PROGRAM AMCI_Assembled_Move_Sample
VAR
FB_Program_Assembled_Move: program_assembled_move_dut;
b_program_assembled_en: BOOL;
b_program_assembled_er: BOOL;
b_program_assembled_dn: BOOL;

FB_run_blend: run_blend_dut;
b_run_blend_en: BOOL;
b_run_blend_er: BOOL;

END_VAR
VAR // added by the converter: edge detectors and wires of the graphical bodies
    _w1, _w2 : BOOL;
END_VAR

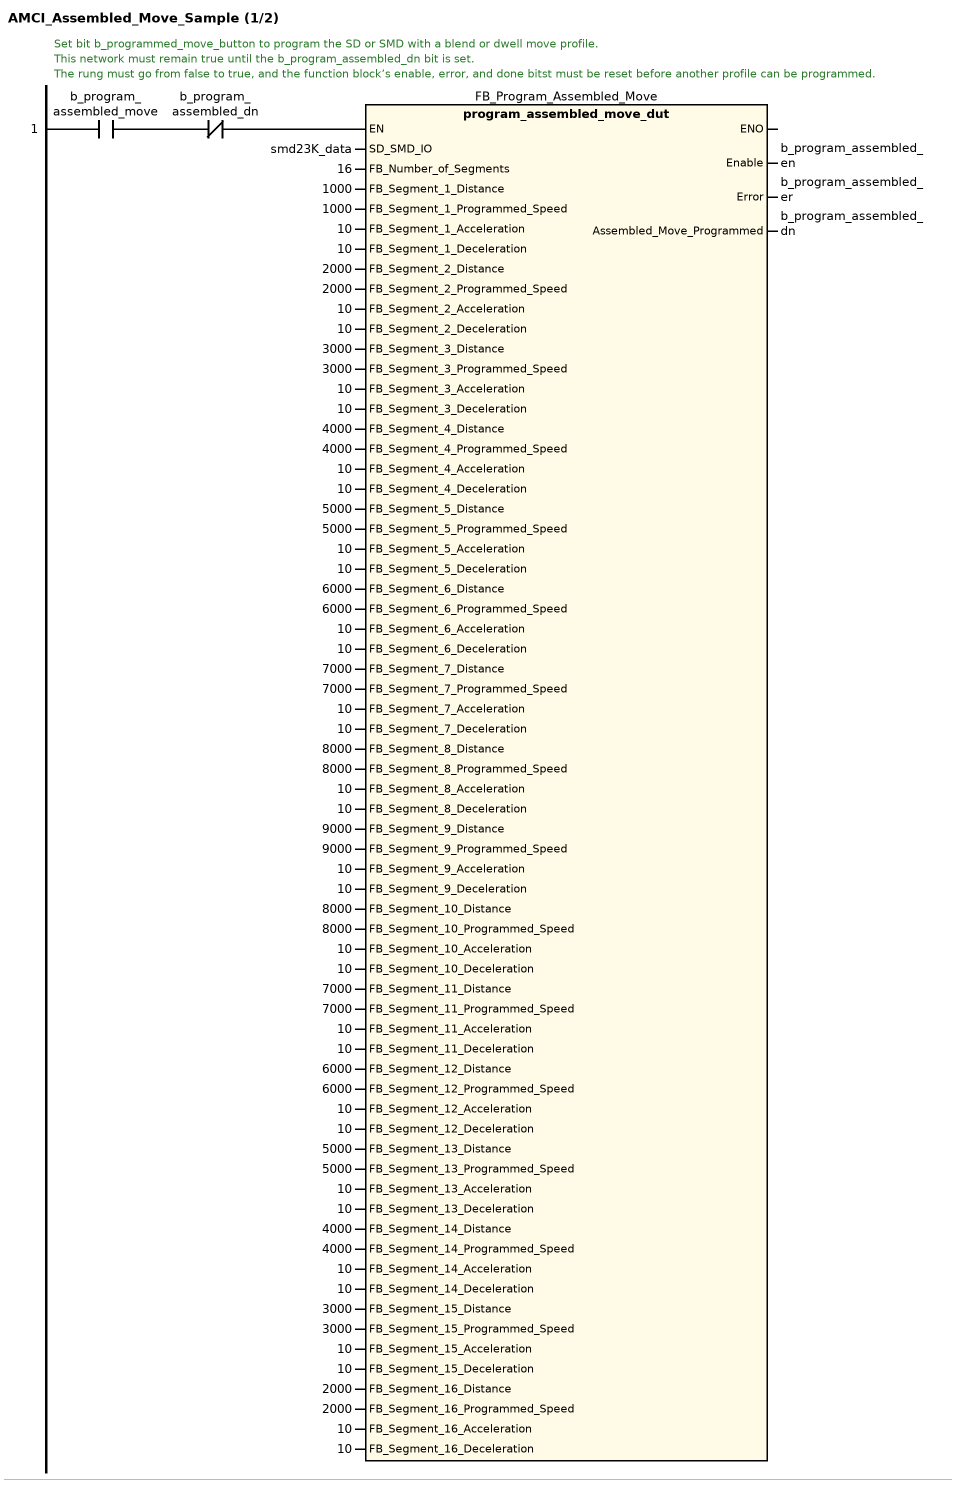
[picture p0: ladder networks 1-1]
// NETWORK 1
// Set bit b_programmed_move_button to program the SD or SMD with a blend or dwell move profile.
//
// This network must remain true until the b_program_assembled_dn bit is set.
//
// The rung must go from false to true, and the function block’s enable, error, and done bitst must be reset before another profile can be programmed.
IF b_program_assembled_move AND NOT b_program_assembled_dn THEN
    FB_Program_Assembled_Move(
        SD_SMD_IO := smd23K_data,
        FB_Number_of_Segments := 16,
        FB_Segment_1_Distance := 1000,
        FB_Segment_1_Programmed_Speed := 1000,
        FB_Segment_1_Acceleration := 10,
        FB_Segment_1_Deceleration := 10,
        FB_Segment_2_Distance := 2000,
        FB_Segment_2_Programmed_Speed := 2000,
        FB_Segment_2_Acceleration := 10,
        FB_Segment_2_Deceleration := 10,
        FB_Segment_3_Distance := 3000,
        FB_Segment_3_Programmed_Speed := 3000,
        FB_Segment_3_Acceleration := 10,
        FB_Segment_3_Deceleration := 10,
        FB_Segment_4_Distance := 4000,
        FB_Segment_4_Programmed_Speed := 4000,
        FB_Segment_4_Acceleration := 10,
        FB_Segment_4_Deceleration := 10,
        FB_Segment_5_Distance := 5000,
        FB_Segment_5_Programmed_Speed := 5000,
        FB_Segment_5_Acceleration := 10,
        FB_Segment_5_Deceleration := 10,
        FB_Segment_6_Distance := 6000,
        FB_Segment_6_Programmed_Speed := 6000,
        FB_Segment_6_Acceleration := 10,
        FB_Segment_6_Deceleration := 10,
        FB_Segment_7_Distance := 7000,
        FB_Segment_7_Programmed_Speed := 7000,
        FB_Segment_7_Acceleration := 10,
        FB_Segment_7_Deceleration := 10,
        FB_Segment_8_Distance := 8000,
        FB_Segment_8_Programmed_Speed := 8000,
        FB_Segment_8_Acceleration := 10,
        FB_Segment_8_Deceleration := 10,
        FB_Segment_9_Distance := 9000,
        FB_Segment_9_Programmed_Speed := 9000,
        FB_Segment_9_Acceleration := 10,
        FB_Segment_9_Deceleration := 10,
        FB_Segment_10_Distance := 8000,
        FB_Segment_10_Programmed_Speed := 8000,
        FB_Segment_10_Acceleration := 10,
        FB_Segment_10_Deceleration := 10,
        FB_Segment_11_Distance := 7000,
        FB_Segment_11_Programmed_Speed := 7000,
        FB_Segment_11_Acceleration := 10,
        FB_Segment_11_Deceleration := 10,
        FB_Segment_12_Distance := 6000,
        FB_Segment_12_Programmed_Speed := 6000,
        FB_Segment_12_Acceleration := 10,
        FB_Segment_12_Deceleration := 10,
        FB_Segment_13_Distance := 5000,
        FB_Segment_13_Programmed_Speed := 5000,
        FB_Segment_13_Acceleration := 10,
        FB_Segment_13_Deceleration := 10,
        FB_Segment_14_Distance := 4000,
        FB_Segment_14_Programmed_Speed := 4000,
        FB_Segment_14_Acceleration := 10,
        FB_Segment_14_Deceleration := 10,
        FB_Segment_15_Distance := 3000,
        FB_Segment_15_Programmed_Speed := 3000,
        FB_Segment_15_Acceleration := 10,
        FB_Segment_15_Deceleration := 10,
        FB_Segment_16_Distance := 2000,
        FB_Segment_16_Programmed_Speed := 2000,
        FB_Segment_16_Acceleration := 10,
        FB_Segment_16_Deceleration := 10,
        Enable => b_program_assembled_en,
        Error => b_program_assembled_er,
        Assembled_Move_Programmed => b_program_assembled_dn); // program_assembled_move_dut
END_IF

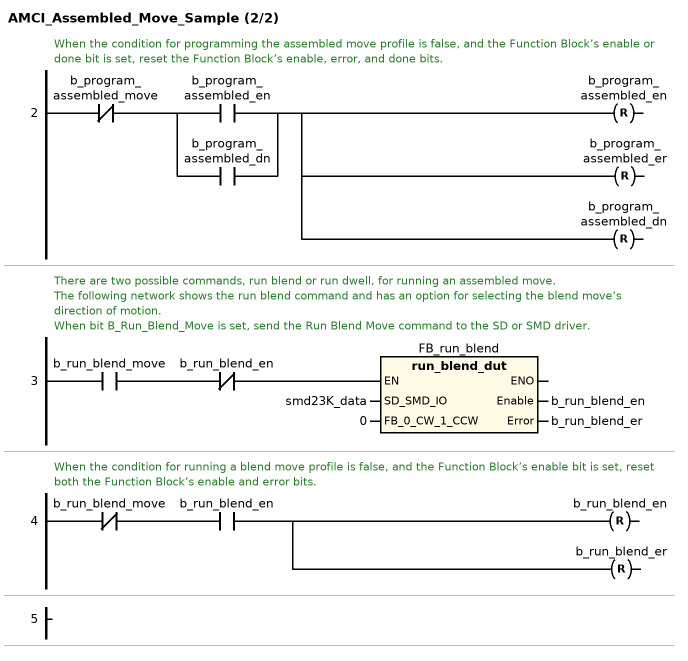
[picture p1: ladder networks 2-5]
// NETWORK 2
// When the condition for programming the assembled move profile is false, and the Function Block’s enable or done bit is set, reset the Function Block’s enable, error, and done bits.
_w1 := NOT b_program_assembled_move AND (b_program_assembled_en OR b_program_assembled_dn);
b_program_assembled_en R= _w1;
b_program_assembled_er R= _w1;
b_program_assembled_dn R= _w1;

// NETWORK 3
// There are two possible commands, run blend or run dwell, for running an assembled move.
//
// The following network shows the run blend command and has an option for selecting the blend move’s direction of motion.
//
// When bit B_Run_Blend_Move is set, send the Run Blend Move command to the SD or SMD driver.
IF b_run_blend_move AND NOT b_run_blend_en THEN
    FB_run_blend(SD_SMD_IO := smd23K_data, FB_0_CW_1_CCW := 0, Enable => b_run_blend_en, Error => b_run_blend_er); // run_blend_dut
END_IF

// NETWORK 4
// When the condition for running a blend move profile is false, and the Function Block’s enable bit is set, reset both the Function Block’s enable and error bits.
_w2 := NOT b_run_blend_move AND b_run_blend_en;
b_run_blend_en R= _w2;
b_run_blend_er R= _w2;

// NETWORK 5

END_PROGRAM
